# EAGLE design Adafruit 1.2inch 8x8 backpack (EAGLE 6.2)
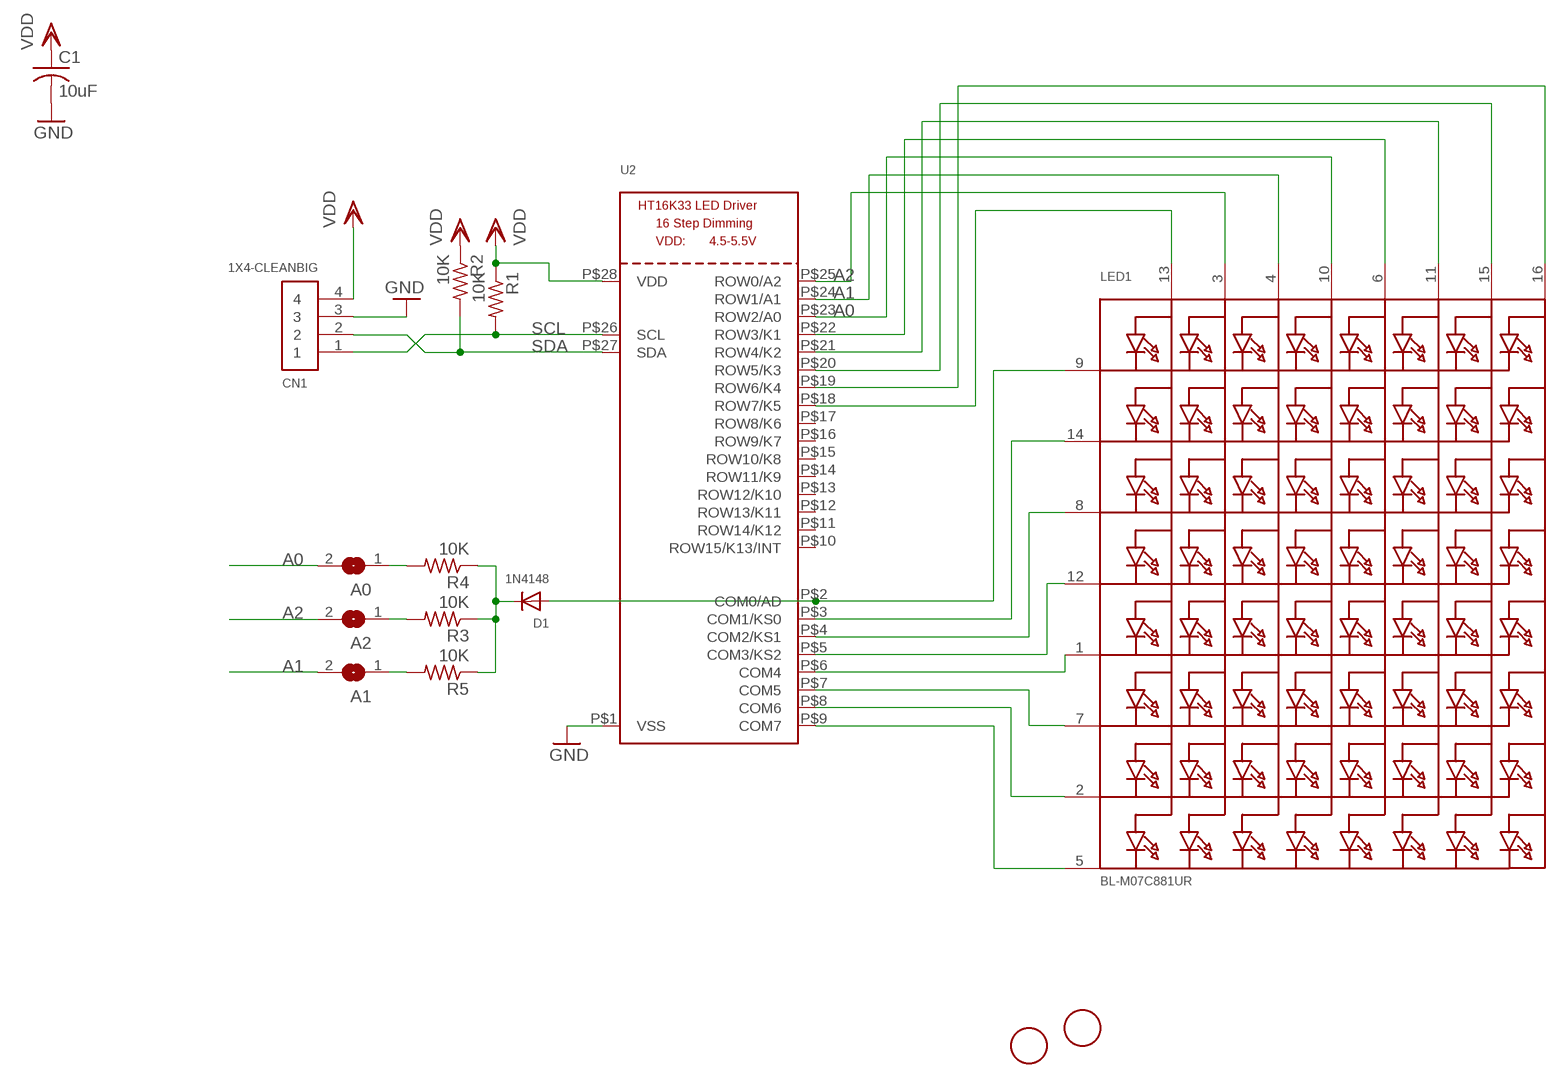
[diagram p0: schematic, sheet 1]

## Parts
A0  SOLDERJUMPERREFLOW_NOPASTE  [SOLDERJUMPER_REFLOW_NOPASTE]
A1  SOLDERJUMPERREFLOW_NOPASTE  [SOLDERJUMPER_REFLOW_NOPASTE]
A2  SOLDERJUMPERREFLOW_NOPASTE  [SOLDERJUMPER_REFLOW_NOPASTE]
C1  10uF  C-USC0805  [C0805]
CN1  1X4-CLEANBIG  [1X04-CLEANBIG]
D1  1N4148  DIODESOD-323F  [SOD-323F]
LED1  BL-M07C881UR  DISP_SEGMENT_8X8_ROWCATHODEM12A881UR  [SEGMENT_BL-M12A881UR]
R1  10K  R-US_R0805  [R0805]
R2  10K  R-US_R0805  [R0805]
R3  10K  R-US_R0805  [R0805]
R4  10K  R-US_R0805  [R0805]
R5  10K  R-US_R0805  [R0805]
U2  HT16K33_SOP28  [SOP28_300MIL]
U$1  FIDUCIAL  [FIDUCIAL_1MM]
U$2  FIDUCIAL  [FIDUCIAL_1MM]

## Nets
A0: A0.2 LED1.10(A4) U2.P$23(ROW2/A0)
A1: A1.2 LED1.4(A3) U2.P$24(ROW1/A1)
A2: A2.2 LED1.3(A2) U2.P$25(ROW0/A2)
GND: C1.2 CN1.3 U2.P$1(VSS)
N$1: LED1.5(K8) U2.P$9(COM7)
N$2: LED1.2(K7) U2.P$8(COM6)
N$3: LED1.7(K6) U2.P$7(COM5)
N$4: LED1.1(K5) U2.P$6(COM4)
N$5: LED1.12(K4) U2.P$5(COM3/KS2)
N$6: LED1.8(K3) U2.P$4(COM2/KS1)
N$7: LED1.14(K2) U2.P$3(COM1/KS0)
N$8: D1.A LED1.9(K1) U2.P$2(COM0/AD)
N$10: A1.1 R5.2
N$12: LED1.6(A5) U2.P$22(ROW3/K1)
N$13: LED1.11(A6) U2.P$21(ROW4/K2)
N$14: D1.C R3.1 R4.1 R5.1
N$16: LED1.13(A1) U2.P$18(ROW7/K5)
N$19: A2.1 R3.2
N$20: A0.1 R4.2
SCL: CN1.1 R1.2 U2.P$26(SCL)
SDA: CN1.2 R2.2 U2.P$27(SDA)
SEG_F: LED1.15(A7) U2.P$20(ROW5/K3)
SEG_G: LED1.16(A8) U2.P$19(ROW6/K4)
VDD: C1.1 CN1.4 R1.1 R2.1 U2.P$28(VDD)
Unconnected: U2.P$10(ROW15/K13/INT) U2.P$11(ROW14/K12) U2.P$12(ROW13/K11) U2.P$13(ROW12/K10) U2.P$14(ROW11/K9) U2.P$15(ROW10/K8) U2.P$16(ROW9/K7) U2.P$17(ROW8/K6)

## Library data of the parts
A0 A1 A2 = microbuilder:SOLDERJUMPER: SMD Solder JUMPER
C1 = rcl:C-US: CAPACITOR, American symbol
CN1 = adafruit:1X4: 4-pin connector
D1 = adafruit:DIODE: Diode
LED1 = microbuilder:DISP_SEGMENT_8X8_ROWCATHODE: 8x8 LED Segment Displays: Row = Cathode 0.7" Red 8X8 Matrix, 1.9mm Round LEDs - BL-M07C881UR 1.2" Red 8x8 Matrix, 3.0mm Round LEDs - BL-M12A881UR 1.2" Red 8x8 Matrix, 3.0mm Square LEDs - BL-M12A883
R1-R5 = adafruit:R-US_: RESISTOR, American symbol
U2 = microbuilder:HT16K33_SOP28
U$1 U$2 = adafruit:FIDUCIAL: For use by pick and place machines to calibrate the vision/machine, 1mm

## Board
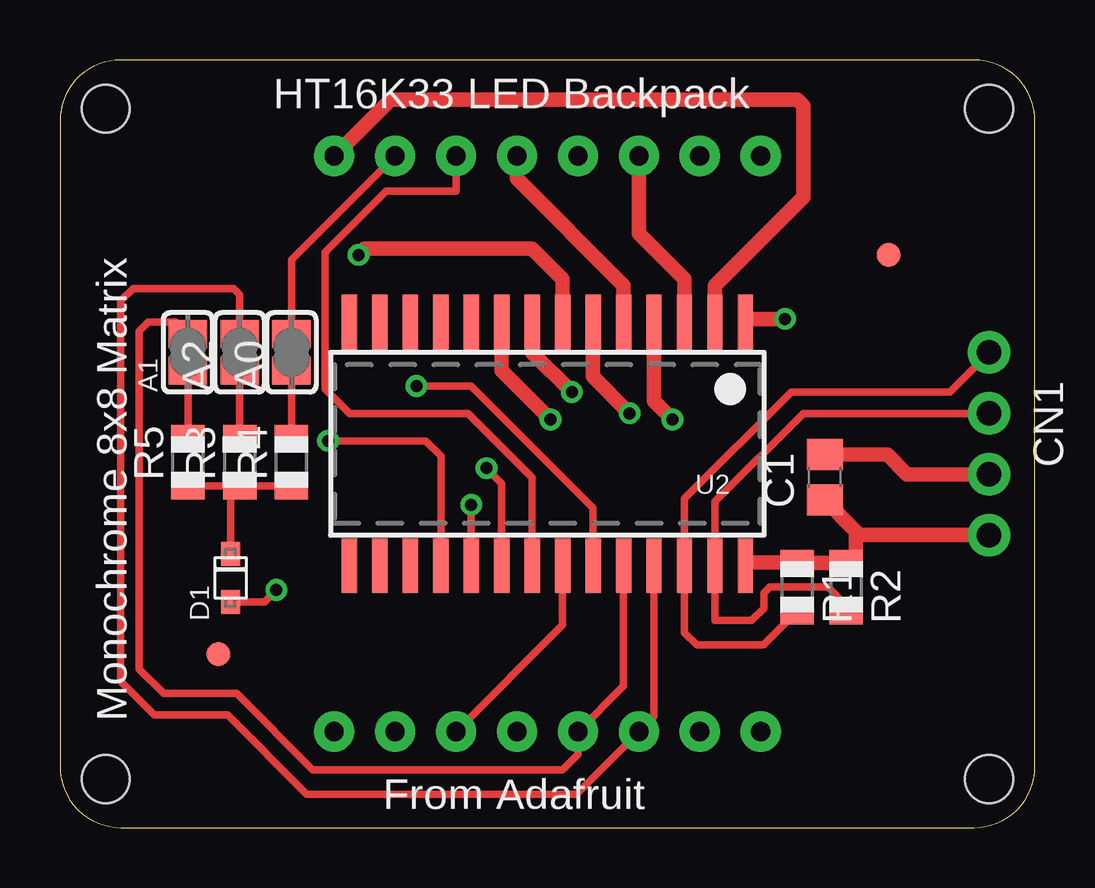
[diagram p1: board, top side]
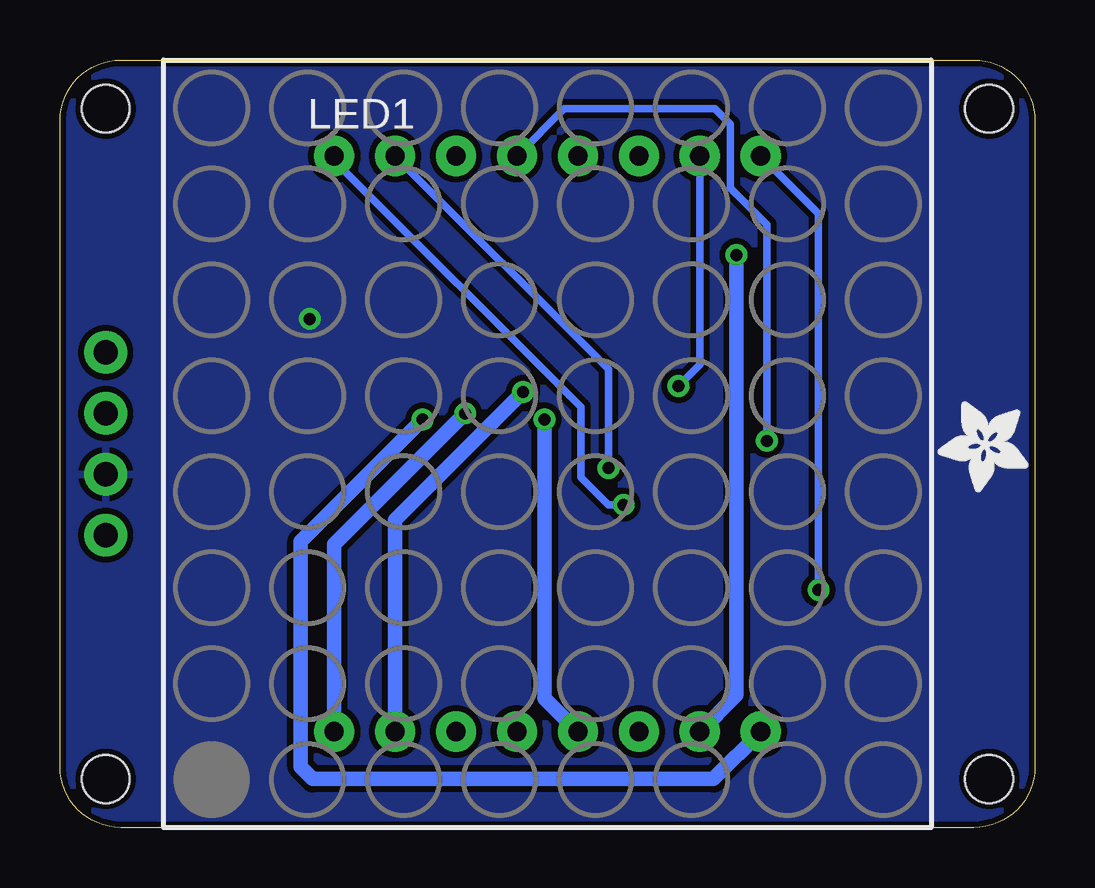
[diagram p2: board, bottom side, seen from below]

Size 40.64 x 32 mm. Coordinates in mm from the lower left corner, seen from the top.
Outline: 0,2.54 arc90 2.54,0 38.1,0 arc90 40.64,2.54 40.64,29.46 arc90 38.1,32 2.54,32 arc90 0,29.46 0,2.54
Copper layers (1*16): Top 0.035mm / dielectric 1.5mm / Bottom 0.035mm
Design rules: minimum track width 10mil, minimum drill 19mil, track to track 10mil, track to pad 10mil, pad to pad 10mil, via to via 10mil, smd to smd 8mil, copper to edge 10mil, drill to drill 8mil, minimum pad ring 10mil, minimum via ring 8mil, stop-mask expansion 4mil, vias tented up to drill 20mil, thermal gap 10mil
Holes 2 mm at 1.91,29.97 1.91,2.03 38.73,29.97 38.73,2.03

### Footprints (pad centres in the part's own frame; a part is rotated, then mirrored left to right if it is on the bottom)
SOLDERJUMPER_REFLOW_NOPASTE = smd 1.168 x 1.6: 1 -0.762,0; 2 0.762,0
C0805 = smd 1.3 x 1.5: 1 -0.95,0; 2 0.95,0
1X04-CLEANBIG = drill 1.016 pad 1.778: 1 -3.81,0; 2 -1.27,0; 3 1.27,0; 4 3.81,0
SOD-323F = smd 1 x 0.8: A -1,0; C 1,0
SEGMENT_BL-M12A881UR = drill 0.8 pad 1.676: 1 -8.89,-12; 2 -6.35,-12; 3 -3.81,-12; 4 -1.27,-12; 5 1.27,-12; 6 3.81,-12; 7 6.35,-12; 8 8.89,-12; 9 8.89,12; 10 6.35,12; 11 3.81,12; 12 1.27,12; 13 -1.27,12; 14 -3.81,12; 15 -6.35,12; 16 -8.89,12
R0805 = smd 1.1 x 1.4: 1 -1,0; 2 1,0
SOP28_300MIL = smd 0.635 x 2.286: P$1 -8.255,-5.08; P$2 -6.985,-5.08; P$3 -5.715,-5.08; P$4 -4.445,-5.08; P$5 -3.175,-5.08; P$6 -1.905,-5.08; P$7 -0.635,-5.08; P$8 0.635,-5.08; P$9 1.905,-5.08; P$10 3.175,-5.08; P$11 4.445,-5.08; P$12 5.715,-5.08; P$13 6.985,-5.08; P$14 8.255,-5.08; P$15 8.255,5.08; P$16 6.985,5.08; P$17 5.715,5.08; P$18 4.445,5.08; P$19 3.175,5.08; P$20 1.905,5.08; P$21 0.635,5.08; P$22 -0.635,5.08; P$23 -1.905,5.08; P$24 -3.175,5.08; P$25 -4.445,5.08; P$26 -5.715,5.08; P$27 -6.985,5.08; P$28 -8.255,5.08
FIDUCIAL_1MM = smd 1 x 1: 1 0,0

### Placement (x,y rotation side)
A0  9.65,19.81 90 top
A1  5.33,19.81 90 top
A2  7.49,19.81 90 top
C1  31.88,14.6 90 top
CN1  38.73,16 270 top
D1  7.11,10.41 90 top
LED1  20.32,16 0 bottom
R1  30.73,10.03 270 top
R2  32.77,10.03 270 top
R3  7.49,15.24 90 top
R4  9.65,15.24 90 top
R5  5.33,15.24 90 top
U2  20.32,16 180 top
U$1  6.6,7.24 270 top
U$2  34.54,23.88 270 top
U$3  [ADAFRUIT_3.5MM]  0.25,17.78 180 bottom

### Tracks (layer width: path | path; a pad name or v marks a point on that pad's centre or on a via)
A0  (via drill 0.5)
  Top 0.305: v14.86,18.41 17.14,18.41 22.23,13.33 U2.P$23 | A0.2 9.65,23.68 LED1.10
  Bottom 0.305: LED1.10 13.97,19.3 v14.86,18.41
A1
  Top 0.305: U2.P$24 23.5,5.91 LED1.4 21.59,3.05 20.96,2.41 10.54,2.41 7.37,5.59 4.32,5.59 3.3,6.6 3.3,20.7 3.68,21.08 4.83,21.08 A1.2
A2
  Top 0.305: U2.P$25 24.77,4.64 LED1.3 21.52,1.4 10.29,1.4 6.98,4.7 3.94,4.7 2.54,6.1 2.54,21.97 3.05,22.48 7.24,22.48 7.49,22.22 A2.2
GND  (via drill 0.5)
  Top 0.61: C1.2 34.48,15.55 35.31,14.73 CN1.3 | U2.P$1 28.7,21.21 v30.23,21.21
  pour Bottom: 40.89,32.38 0,32.38 0,-0.25 40.89,-0.25
N$1  (via drill 0.5)
  Top 0.61: U2.P$9 18.41,19.05 v20.45,17.02
  Bottom 0.61: v20.45,17.02 20.45,5.4 LED1.5
N$2  (via drill 0.5)
  Top 0.61: U2.P$8 19.68,19.81 v21.34,18.16
  Bottom 0.61: v21.34,18.16 26.67,12.83 LED1.2
N$3  (via drill 0.5)
  Top 0.61: U2.P$7 20.96,22.86 19.68,24.13 12.7,24.13 v12.45,23.88
  Bottom 0.61: v12.45,23.88 12.45,5.53 LED1.7
N$4  (via drill 0.5)
  Top 0.61: U2.P$6 22.23,18.8 v23.75,17.27
  Bottom 0.61: v23.75,17.27 29.21,11.81 LED1.1
N$5
  Top 0.61: U2.P$5 23.5,22.61 19.05,27.05 LED1.12
N$6  (via drill 0.5)
  Top 0.61: v25.53,17.02 24.77,17.78 U2.P$4
  Bottom 0.61: LED1.8 13.4,2.03 30.1,2.03 30.61,2.54 30.61,11.94 v25.53,17.02
N$7
  Top 0.61: LED1.14 24.13,24.77 26.04,22.86 U2.P$3
N$8  (via drill 0.5)
  Top 0.305: D1.A 8.53,9.41 v9.02,9.91
  Top 0.61: U2.P$2 27.3,22.61 30.99,26.29 30.99,30.1 30.73,30.35 13.78,30.35 LED1.9
  Bottom 0.305: v9.02,9.91 9.02,25.59 LED1.9
N$10
  Top 0.305: A1.1 R5.2
N$12
  Top 0.305: U2.P$22 20.96,8.45 LED1.6
N$13
  Top 0.305: LED1.11 16.51,26.54 13.59,26.54 11.05,24 11.05,18.29 12.06,17.27 17.02,17.27 19.68,14.6 U2.P$21
N$14
  Top 0.305: D1.C 7.11,14.24 R3.1 | R3.1 R4.1 | R5.1 R3.1
N$16  (via drill 0.5)
  Top 0.305: U2.P$18 15.88,15.49 15.24,16.13 v11.18,16.13
  Bottom 0.305: LED1.13 19.62,29.97 13.34,29.97 12.7,29.34 12.7,26.67 11.18,25.15 v11.18,16.13
N$19
  Top 0.305: R3.2 A2.1
N$20
  Top 0.305: R4.2 A0.1
SCL
  Top 0.305: R1.2 29.32,7.62 26.54,7.62 26.04,8.13 U2.P$26 26.04,13.72 30.48,18.16 37.08,18.16 CN1.1
SDA
  Top 0.305: R2.2 32.77,9.27 32,10.03 29.59,10.03 29.34,9.78 29.34,9.14 28.83,8.64 27.3,8.64 U2.P$27 27.3,13.59 30.99,17.27 CN1.2
SEG_F  (via drill 0.5)
  Top 0.305: U2.P$20 18.41,14.35 v17.78,14.99
  Bottom 0.305: v17.78,14.99 17.78,19.11 LED1.15
SEG_G  (via drill 0.5)
  Top 0.305: v17.14,13.46 U2.P$19
  Bottom 0.305: LED1.16 29.21,27.81 18.92,17.53 18.92,14.6 17.78,13.46 v17.14,13.46
VDD
  Top 0.61: C1.1 33.18,12.35 | 33.18,12.35 33.34,12.19 CN1.4 | U2.P$28 28.7,11.05 30.1,11.05 30.12,11.03 R1.1 R2.1 33.18,11.45 33.18,12.35

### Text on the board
tPlace: HT16K33 LED Backpack | Monochrome 8x8 Matrix | From Adafruit
tDocu: SCL | SDA | GND | VCC | A2 | A1 | A0
bDocu: C | D | - | +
